(* Logix 5000 AddOnInstructionDefinition export TeNod4TBlocFilters; software revision 28.00 *)

ADD_ON_INSTRUCTION TeNod4TBlocFilters   (* revision 1.1, vendor Scaime *)
VAR_IN_OUT
   Datas : TeNod4TDatas; {required}
END_VAR
VAR_INPUT
   Read : BOOL; {visible}
   Write : BOOL; {visible}
END_VAR
VAR_OUTPUT
   InProgress : BOOL; {visible}
   Done : BOOL; {visible}
   Error : BOOL; {visible}
END_VAR
VAR
   IntRead : BOOL; {access None}
   IntWrite1 : BOOL; {access None}
   IntWrite2 : BOOL; {access None}
END_VAR

ROUTINE Logic   (* ladder *)
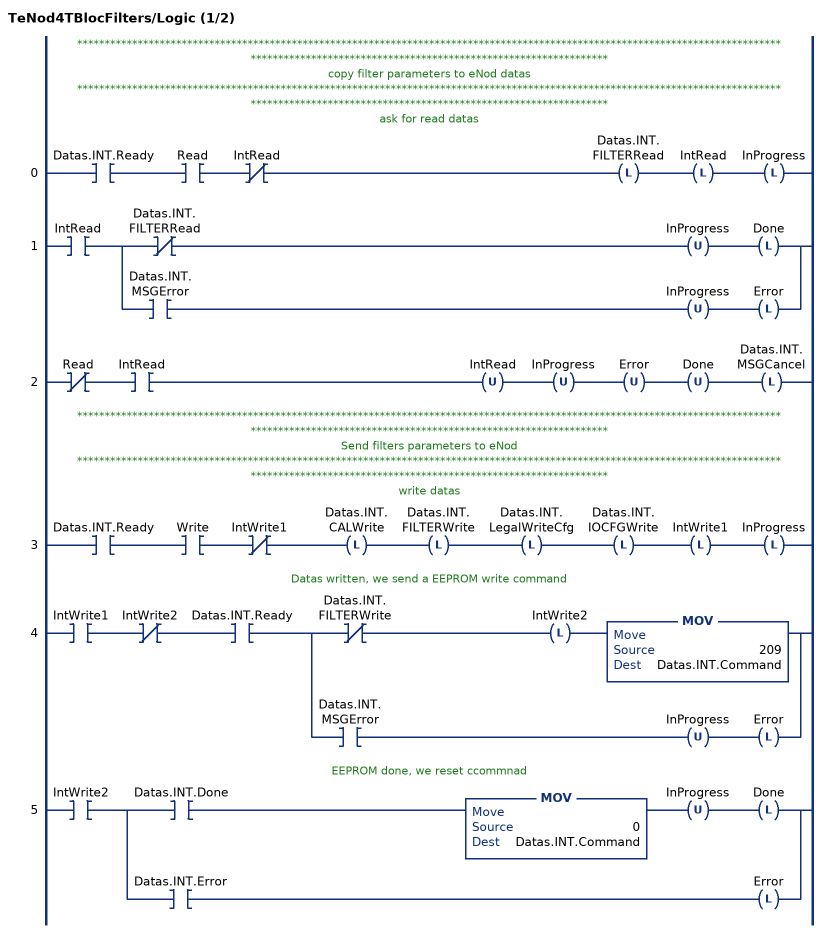
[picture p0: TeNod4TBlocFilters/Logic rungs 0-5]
   // *************************************************************************************************************************************************************************************************
   // copy filter parameters to eNod datas
   // *************************************************************************************************************************************************************************************************
   // ask for read datas
   0: XIC(Datas.INT.Ready)XIC(Read)XIO(IntRead)OTL(Datas.INT.FILTERRead)OTL(IntRead)OTL(InProgress);
   1: XIC(IntRead)[XIO(Datas.INT.FILTERRead) OTU(InProgress) OTL(Done) ,XIC(Datas.INT.MSGError) OTU(InProgress) OTL(Error) ];
   2: XIO(Read)XIC(IntRead)OTU(IntRead)OTU(InProgress)OTU(Error)OTU(Done)OTL(Datas.INT.MSGCancel);
   // *************************************************************************************************************************************************************************************************
   // Send filters parameters to eNod
   // *************************************************************************************************************************************************************************************************
   // write datas
   3: XIC(Datas.INT.Ready)XIC(Write)XIO(IntWrite1)OTL(Datas.INT.CALWrite)OTL(Datas.INT.FILTERWrite)OTL(Datas.INT.LegalWriteCfg)OTL(Datas.INT.IOCFGWrite)OTL(IntWrite1)OTL(InProgress);
   // Datas written, we send a EEPROM write command
   4: XIC(IntWrite1)XIO(IntWrite2)XIC(Datas.INT.Ready)[XIO(Datas.INT.FILTERWrite) OTL(IntWrite2) MOV(209,Datas.INT.Command) ,XIC(Datas.INT.MSGError) OTU(InProgress) OTL(Error) ];
   // EEPROM done, we reset ccommnad
   5: XIC(IntWrite2)[XIC(Datas.INT.Done) MOV(0,Datas.INT.Command) OTU(InProgress) OTL(Done) ,XIC(Datas.INT.Error) OTL(Error) ];
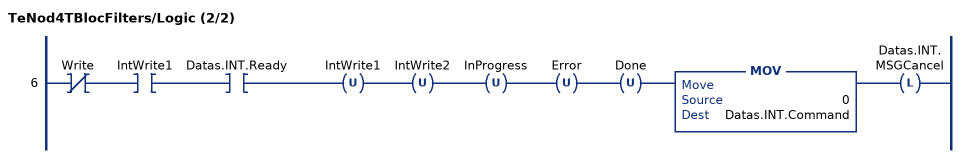
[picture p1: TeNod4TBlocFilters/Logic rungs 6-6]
   6: XIO(Write)XIC(IntWrite1)XIC(Datas.INT.Ready)OTU(IntWrite1)OTU(IntWrite2)OTU(InProgress)OTU(Error)OTU(Done)MOV(0,Datas.INT.Command)OTL(Datas.INT.MSGCancel);
END_ROUTINE
END_ADD_ON_INSTRUCTION
